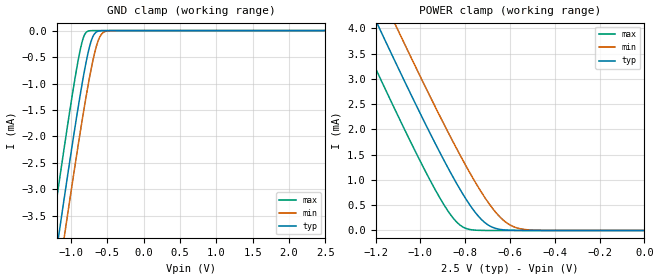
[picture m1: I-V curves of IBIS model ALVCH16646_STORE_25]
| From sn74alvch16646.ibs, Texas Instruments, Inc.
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[Model]   ALVCH16646_STORE_25
Model_type  Input
Vinl=0.7
Vinh=1.7
| variable   typ   min   max
C_comp   1.58pF   1.44pF   1.95pF
[Temperature Range]   40   100   -40
| Ambient temperature   25   85   -40
[Voltage range]   2.5   2.3   2.7
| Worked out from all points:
|   GND clamp passes 1 mA (typ) near -0.85 V on its own axis
|   POWER clamp passes 1 mA (typ) near -0.85 V on its own axis
[GND Clamp]
| ALVCH16646_STORE_25
|   Voltage   I(typ)   I(min)   I(max)
-2.5V     -16.88mA   -17.58mA   -15.98mA
-1.285V   -4.967mA   -5.705mA   -4.014mA
-1.25V    -4.634mA   -5.373mA   -3.679mA
-1.155V   -3.736mA   -4.476mA   -2.78mA
-1.075V   -2.991mA   -3.73mA    -2.037mA
-880mV    -1.265mA   -1.975mA   -406.2uA
-830mV    -866.7uA   -1.551mA   -133.3uA
-780mV    -510.2uA   -1.147mA   -20.22uA
-710mV    -148.5uA   -636.7uA   -739.2nA
-640mV    -18.77uA   -246.3uA   -24.69nA
-515mV    -217.6nA   -11.23uA   -63.37pA
2.5V      4.712pA    817.5pA    4.189pA
[POWER Clamp]
| ALVCH16646_STORE_25
|   Voltage   I(typ)   I(min)   I(max)
-2.5V     16.88mA    17.58mA    15.98mA
-1.3V     5.111mA    5.849mA    4.158mA
-1.255V   4.681mA    5.42mA     3.727mA
-1.18V    3.971mA    4.711mA    3.015mA
-1.11V    3.316mA    4.055mA    2.36mA
-940mV    1.776mA    2.501mA    856.4uA
-845mV    982.9uA    1.676mA    200.1uA
-795mV    611.2uA    1.266mA    38.41uA
-725mV    207uA      738.7uA    1.527uA
-625mV    11.21uA    186.8uA    11.91nA
-510mV    181.6nA    9.688uA    51.12pA
-31.15fV  4.712pA    6.41pA     4.886pA
